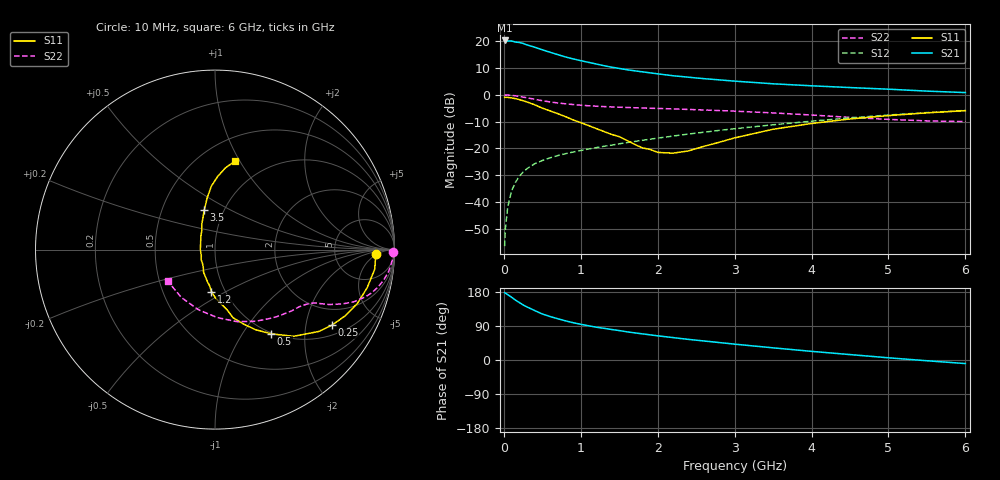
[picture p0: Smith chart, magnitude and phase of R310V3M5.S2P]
! SIEMENS Small Signal Semiconductors
! BFR181
! Si NPN RF Bipolar Junction Transistor in SOT23
! VCE = 10 V  IC = 3.5 mA
! Common Emitter S-Parameters:  May  1996
# GHz  S  MA  R  50
!  f  S11  S21  S12  S22
! GHz  MAG  ANG  MAG  ANG  MAG  ANG  MAG  ANG
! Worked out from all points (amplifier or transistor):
!   36 points, 10 MHz to 6 GHz, reference 50 ohm
!   highest |S21| = 20.3 dB at 10 MHz (marker M1)
!   |S21| within 3 dB of that: start of sweep to 450.6 MHz
!   unconditionally stable (mu >= 1): 1.369 GHz to 3.301 GHz
!   at 250 MHz: K = 0.33, MSG = 24.0 dB, |S12| = -28.9 dB
!   at 1.4 GHz: K = 1.01, MAG = 14.0 dB, |S12| = -18.8 dB
!   at 6 GHz: K = 0.86, MSG = 3.3 dB, |S12| = -5.8 dB
!   S11 on the Smith chart (normalised r, x): 10 MHz: 18, -4; 250 MHz: 1.33, -2.81; 500 MHz: 0.99, -1.35; 1.2 GHz: 0.86, -0.43; 3.5 GHz: 0.81, +0.37; 6 GHz: 0.72, +0.96
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0.01  0.8977 -1.5  10.32 177.8  0.0015 93.0  0.993 -0.7
0.02  0.8956 -2.7  10.08 176.4  0.0032 88.3  0.9876 -1.4
0.05  0.8966 -7.0  10.14 172.5  0.0079 86.0  0.9895 -3.5
0.1  0.8739 -14.1  10.07 165.7  0.0161 80.8  0.9766 -6.9
0.15  0.8487 -20.6  9.654 158.2  0.0231 78.1  0.9569 -10.0
0.2  0.8143 -26.9  9.461 151.7  0.0302 74.5  0.9333 -12.8
0.25  0.7749 -33.0  9.087 145.4  0.036 71.6  0.9063 -15.4
0.3  0.7361 -38.3  8.533 140.1  0.0418 70.1  0.8789 -17.4
0.4  0.6514 -47.9  7.731 130.6  0.0516 65.9  0.8264 -20.6
0.5  0.5635 -56.3  6.913 121.4  0.0594 63.5  0.7757 -22.9
0.6  0.5016 -63.0  6.223 114.8  0.0666 61.9  0.7349 -24.5
0.8  0.392 -75.2  5.095 103.4  0.0796 60.0  0.6792 -26.5
0.9  0.3406 -78.8  4.677 98.4  0.0855 59.7  0.658 -27.2
1.1  0.2671 -89.8  4.035 90.4  0.0975 60.1  0.6245 -28.5
1.2  0.2346 -94.8  3.755 86.6  0.1032 60.3  0.6121 -29.3
1.6  0.141 -117.0  2.931 74.4  0.1282 60.3  0.5806 -32.4
2.2  0.0814 179.4  2.268 59.1  0.17 59.7  0.5458 -38.9
3  0.1571 118.0  1.798 41.8  0.2327 56.3  0.4952 -50.4
3.5  0.2276 105.3  1.604 32.1  0.2758 52.8  0.4592 -60.4
4.5  0.3539 93.3  1.364 14.3  0.3706 43.6  0.3788 -88.1
5.5  0.4604 82.6  1.171 -2.0  0.466 31.8  0.326 -125.1
6  0.5054 77.2  1.1 -9.4  0.5106 25.0  0.3166 -145.9
